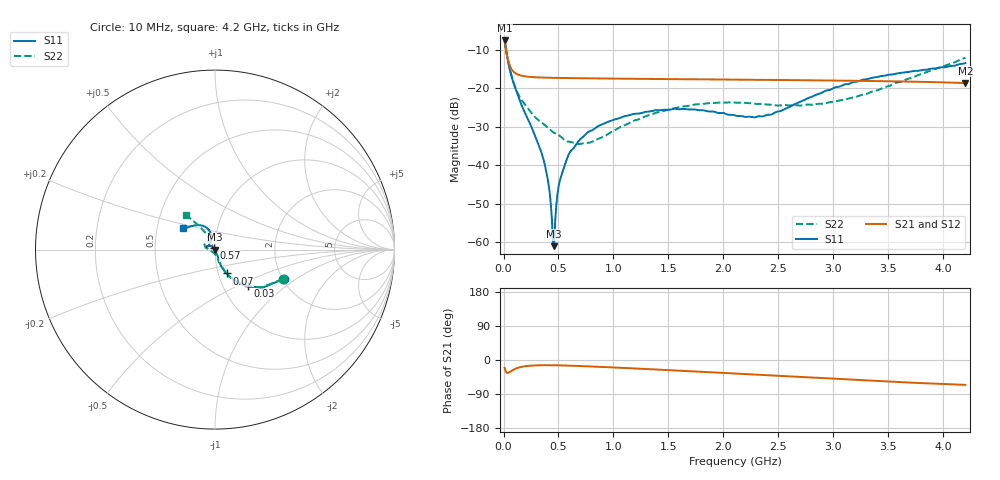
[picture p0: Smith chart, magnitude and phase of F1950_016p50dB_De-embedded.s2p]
! Integrated Device Technology
! Corporate Headquarters
! 6024 Silver Creek Valley Road
! San Jose, CA 95138  USA
! Phone:  1-408-284-8200
! Toll Free:  1-800-223-1366
! Webpage:  http://www.idt.com/
! Timing and RF Division
! 515 Groton Road, Suite 102
! Westford, MA 01886-6024
! Device:  F1950
! Description: 7-bit 0.25 dB Digital Step Attenuator
! Frequency:  150.0 -  4000.00 MHz
! Package:  4x4 mm Thin QFN Plastic Package: 24 pin
! Ports:  2 RF, 12 DC
!  Pin  1  = D0
!  Pin  2  = VDD
!  Pin  3  = Vmode
!  Pin  4  = GND
!  Pin  5  = RF1  =  Port 1
!  Pin  6  = GND
!  Pin  7  = GND
!  Pin  8  = GND
!  Pin  9  = GND
!  Pin 10  = GND
!  Pin 11  = GND
!  Pin 12  = GND
!  Pin 13  = GND
!  Pin 14  = RF2  =  Port 2
!  Pin 15  = GND
!  Pin 16  = LE
!  Pin 17  = CLK
!  Pin 18  = DATE
!  Pin 19  = D6
!  Pin 20  = D5
!  Pin 21  = D4
!  Pin 22  = D3
!  Pin 23  = D2
!  Pin 24  = D1
! State:  66
! Atten State:  16.50 dB
! Voltage:  +5.00 Volts
! Current:  Not Measured mA
! Data:  The device was measured on a the F195X evaluation board which has
!  individual transmission lines to the RF pins.  Data was collected
!  using a calibrated network analyzer.  The evaluation board was
!  de-embedded using a TRL calibration technique.
!  The reference plane is the edge of the package pin.
! Misc:  Board 2019
!  Action Tracker AT0250
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# GHz S dB R 50
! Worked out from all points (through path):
!   420 points, 10 MHz to 4.2 GHz, reference 50 ohm
!   highest |S21| = -7.59 dB at 10 MHz (marker M1); lowest = -18.6 dB at 4.2 GHz (marker M2)
!   group delay of S21, straight-line fit = 36.7 ps
!   lowest |S11| = -61.0 dB at 460 MHz (marker M3), VSWR 1.00, Z = 49.9 + j0.0183 ohm
!   |S11| at or under -10 dB: 23.38 MHz to end of sweep
!   |S22| runs from -34.5 to -7.7 dB; largest |S21 - S12| = 0.0002
!   S11 on the Smith chart (normalised r, x): 10 MHz: 2.04, -0.80; 30 MHz: 1.31, -0.58; 70 MHz: 1.09, -0.30; 570 MHz: 0.98, +0.02; 4.2 GHz: 0.68, +0.17
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0.01  -7.59 -23.0  -7.59 -20.5  -7.58 -20.5  -7.72 -23.7
0.03  -11.20 -48.0  -11.20 -33.8  -11.19 -33.8  -11.22 -48.3
0.07  -16.63 -64.2  -14.91 -29.1  -14.91 -29.1  -16.42 -63.9
0.16  -24.03 -70.6  -16.70 -18.3  -16.70 -18.3  -22.82 -72.1
0.36  -38.11 -65.1  -17.22 -13.7  -17.22 -13.7  -29.15 -80.9
0.41  -45.00 -69.6  -17.26 -13.7  -17.26 -13.7  -30.41 -82.7
0.44  -53.94 -83.5  -17.28 -13.8  -17.28 -13.8  -31.16 -86.2
0.46  -60.95 168.2  -17.29 -13.9  -17.29 -13.9  -31.54 -89.2
0.47  -54.46 139.8  -17.30 -13.9  -17.30 -13.9  -31.68 -90.7
0.49  -47.58 131.5  -17.31 -14.0  -17.31 -14.0  -31.96 -92.9
0.51  -44.19 132.3  -17.32 -14.1  -17.31 -14.2  -32.29 -94.3
0.57  -38.83 131.0  -17.34 -14.6  -17.34 -14.6  -33.70 -103.1
0.61  -36.34 133.7  -17.36 -15.0  -17.36 -15.0  -33.90 -110.6
0.71  -32.92 136.3  -17.39 -16.0  -17.39 -16.0  -34.34 -128.3
0.99  -28.28 147.0  -17.48 -19.6  -17.48 -19.6  -31.22 -169.9
1.41  -25.69 163.3  -17.59 -25.4  -17.59 -25.4  -26.16 168.3
1.73  -25.46 168.9  -17.66 -30.0  -17.66 -30.0  -24.26 159.7
2.11  -27.09 158.6  -17.75 -35.8  -17.75 -35.9  -23.72 150.6
2.43  -26.83 126.9  -17.83 -40.6  -17.83 -40.6  -24.24 141.2
2.81  -22.11 105.6  -17.92 -46.5  -17.92 -46.5  -24.26 126.7
3.51  -16.47 117.6  -18.17 -57.1  -18.17 -57.1  -19.37 120.0
4.2  -13.47 146.0  -18.64 -65.6  -18.64 -65.7  -12.06 129.9
